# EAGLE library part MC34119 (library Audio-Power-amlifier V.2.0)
The MC34119 is a MOTOROLA low power audio amplifier intergrated circuit intended (primarily) for telephone applications, such as in speakerphones. It provides differential speaker outputs to maximize output swing at low supply voltages (2.0 V minimum). Coupling capacitors to the speaker are not required. Open loop gain is 80 dB, and the closed loop gain is set with two external resistors. A Chip Disable pin permits powering down and/or muting the input signal.
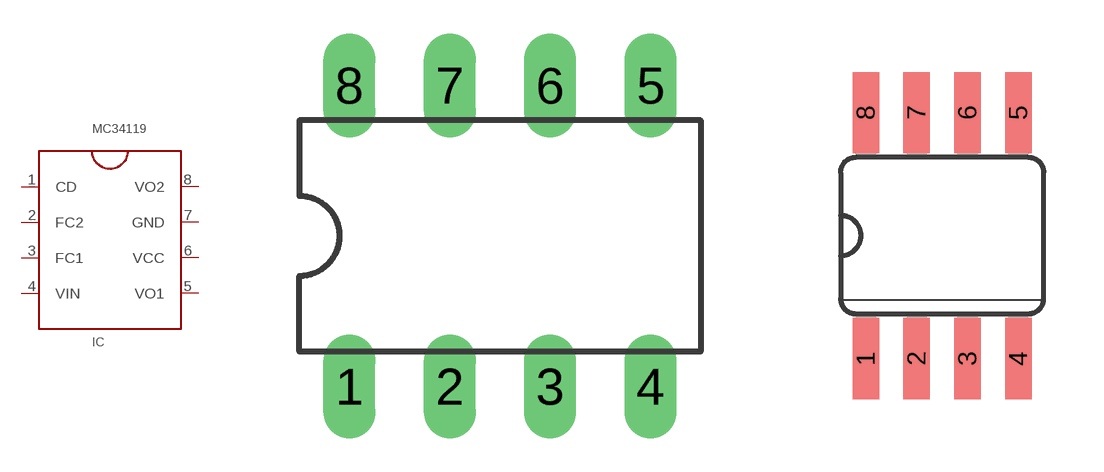
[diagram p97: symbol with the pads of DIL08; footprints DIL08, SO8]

Designator prefix IC

## MC34119MC34119P  [DIL08]
1  CD  in
2  FC2
3  FC1
4  VIN  in
5  VO1  out
6  VCC  pwr
7  GND  pwr
8  VO2  out

## MC34119MC34119D  [SO8]
Pads as for DIL08

## MC34119MC34119DTB  [TSSOP8]
Pads as for DIL08

## Footprint DIL08 (pad centres in mm)
Dual In Line Package
drill 0.813 pad 1.27 long: 1 -3.81,-3.81; 2 -1.27,-3.81; 3 1.27,-3.81; 4 3.81,-3.81; 5 3.81,3.81; 6 1.27,3.81; 7 -1.27,3.81; 8 -3.81,3.81

## Footprint SO8 (pad centres in mm)
smd 0.66 x 2.032: 1 -1.905,-3.073; 2 -0.635,-3.073; 3 0.635,-3.073; 4 1.905,-3.073; 5 1.905,3.073; 6 0.635,3.073; 7 -0.635,3.073; 8 -1.905,3.073

## Footprint TSSOP8 (pad centres in mm)
Thin Shrink Small Outline Package package type ST
smd 0.35 x 1.2: 1 -0.975,-2.925; 2 -0.325,-2.925; 3 0.325,-2.925; 4 0.975,-2.925; 5 0.975,2.925; 6 0.325,2.925; 7 -0.325,2.925; 8 -0.975,2.925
